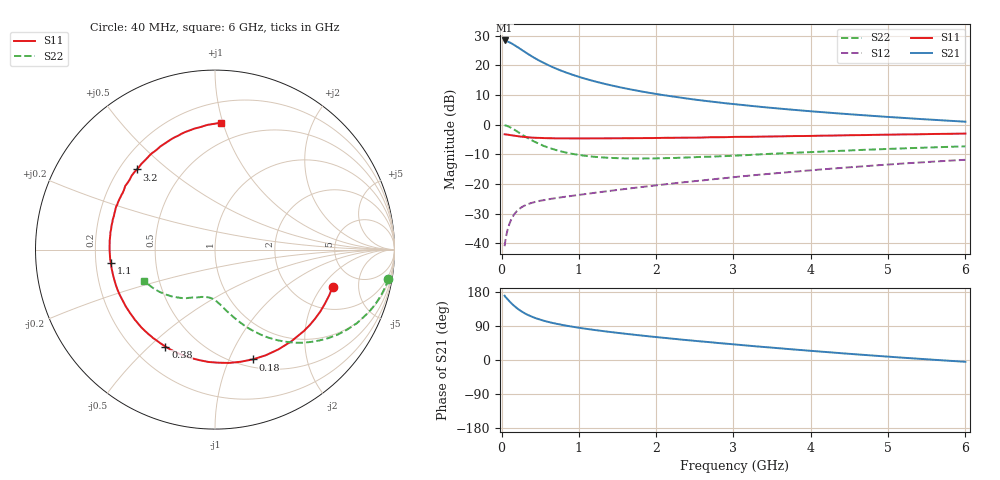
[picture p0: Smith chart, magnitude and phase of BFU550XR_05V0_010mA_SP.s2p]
! Filename:  P:\Prog\Test\Noise\ATS_data\Testdata_Net\03 Spar\BFU550XR_APG2013_45_C05_05p0V_010mA_SP_CM01_D.s2p
! Date/Time: Tue 06/Aug/2013 14:38:16
! BFU550XR_APG2013_45_C05_05p0V_1to35mA_SP_CM01_Bias5_R.s2p
! MDIF S-parameter v. bias file
! BFU550XR_APG2013_45_C05_05p0V_1to35mA_SP_CM01
! Date/time Fri Aug 02 14:46:46 2013
! VAR V_out= 5.0000
! VAR I_out= 10.0000
! VAR V_in= 0.8240
! VAR I_in= 0.1103
! Device data file deembeded for feedlines and parallel
! Original file: \03 Spar\BFU550XR_APG2013_45_C05_05p0V_010mA_SP_CM01_R.s2p
! Feed-files: PR006V01_02082013_Feed1.s2p, PR006V01_02082013_Feed2.s2p
! Parallel-file: PR006V01_02082013_Par.s2p
# MHz S MA R 50
!  Freq-MHz  S11-mag  S11-arg  S21-mag  S21-arg  S12-mag  S12-arg  S22-mag  S22-arg
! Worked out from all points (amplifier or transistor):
!   98 points, 40 MHz to 6 GHz, reference 50 ohm
!   highest |S21| = 28.4 dB at 40 MHz (marker M1)
!   |S21| within 3 dB of that: start of sweep to 251.2 MHz
!   unconditionally stable (mu >= 1): 1.904 GHz to 3.941 GHz
!   at 300 MHz: K = 0.28, MSG = 26.0 dB, |S12| = -27.3 dB
!   at 1.6 GHz: K = 0.94, MSG = 17.0 dB, |S12| = -21.7 dB
!   at 6 GHz: K = 0.87, MSG = 6.4 dB, |S12| = -11.9 dB
!   S11 on the Smith chart (normalised r, x): 40 MHz: 3.25, -2.57; 180 MHz: 0.58, -1.22; 380 MHz: 0.33, -0.56; 1.1 GHz: 0.26, -0.06; 3.2 GHz: 0.27, +0.40; 6 GHz: 0.35, +0.98
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40  0.6878 -17.6  26.39 169.6  0.008882 81.6  0.9786 -9.6
50  0.6854 -21.8  26.25 166.6  0.01106 80.1  0.973 -12.0
80  0.6776 -34.5  25.28 159.9  0.01706 74.2  0.9424 -19.0
120  0.6647 -50.4  23.94 151.2  0.02415 67.4  0.8906 -27.4
140  0.6587 -57.6  23.13 147.2  0.02721 64.5  0.8601 -31.3
180  0.6468 -71.1  21.45 140.0  0.03259 59.1  0.7999 -38.1
220  0.6363 -83.0  19.91 133.6  0.03684 55.0  0.7416 -43.9
280  0.6222 -97.9  17.63 125.6  0.04178 50.0  0.6616 -51.3
320  0.6148 -106.6  16.32 121.1  0.04428 47.6  0.6149 -55.3
380  0.6066 -117.1  14.55 115.4  0.04734 44.9  0.555 -60.3
500  0.5971 -133.2  11.83 106.6  0.05192 41.8  0.4659 -67.8
650  0.5894 -147.4  9.503 98.3  0.05619 40.5  0.3924 -74.4
800  0.5873 -157.7  7.899 92.0  0.06008 40.5  0.3466 -79.4
1050  0.5857 -170.4  6.136 83.6  0.06639 41.9  0.3016 -85.6
1100  0.585 -172.5  5.87 82.1  0.06776 42.2  0.296 -86.8
1500  0.5888 173.5  4.364 71.6  0.07907 44.5  0.272 -94.3
2050  0.5965 159.0  3.217 59.5  0.09599 46.5  0.2708 -103.0
3100  0.6229 136.3  2.159 39.5  0.1338 46.7  0.3031 -117.7
3200  0.6236 134.3  2.093 37.7  0.1376 46.4  0.3073 -118.9
4100  0.6501 118.0  1.644 22.6  0.1738 42.8  0.3486 -131.1
5200  0.6838 99.7  1.299 6.0  0.2211 35.9  0.3975 -145.6
6000  0.7071 87.5  1.123 -4.8  0.255 29.8  0.4307 -156.2
